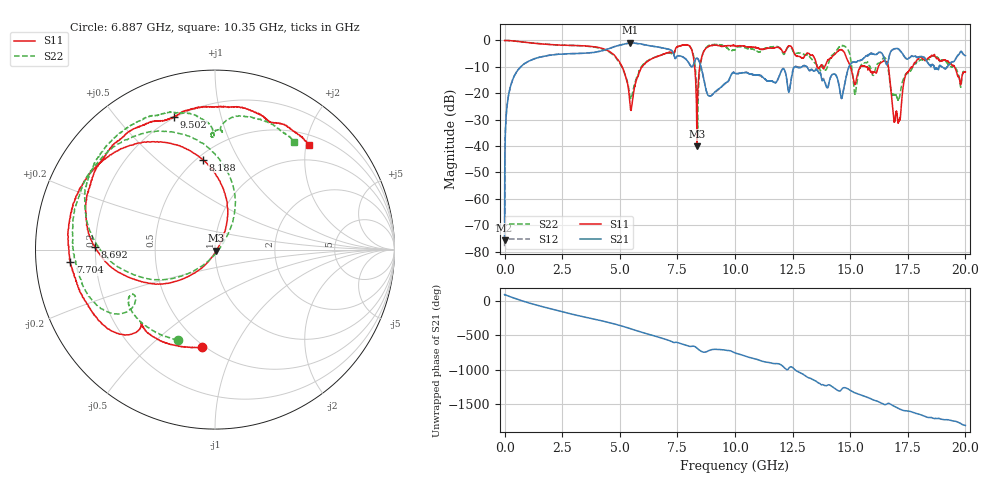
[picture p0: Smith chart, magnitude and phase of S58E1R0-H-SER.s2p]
!{S58E1R0}
!Johanson Technology Inc.
!www.johansontechnology.com
!Test Board Conditions:
!Substrate Type  RO4350B
!Substrate Thickness  60 mil
!Substrate Dk  3.66
!TL Type: GCPW
!TL Trace Width  115 mil
!TL Gap  52 mil
!Electrode orientation  Horizontal
!DUT TOPOLOGY	SERIES
!Mounting Pad LxW  55x428 mil
! Created Tue Apr 13 21:45:22 2021
# hz S ma R 50
! 2 Port Network Data from SP1.SP block
! freq  magS11  angS11  magS21  angS21  magS12  angS12  magS22  angS22
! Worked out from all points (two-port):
!   20001 points, 300 kHz to 20 GHz, reference 50 ohm
!   highest |S21| = -0.87 dB at 5.44 GHz (marker M1); lowest = -75.7 dB at 300 kHz (marker M2)
!   |S21| within 3 dB of the highest: 4.24 GHz to 7.264 GHz (3.024 GHz wide, 52.6 % of centre); 16.79 GHz to 17.17 GHz (381.5 MHz wide, 2.25 % of centre)
!   lowest |S11| = -40.1 dB at 8.347 GHz (marker M3), VSWR 1.02, Z = 50.8 - j0.539 ohm
!   |S11| at or under -10 dB: 5.105 GHz to 5.965 GHz (860.2 MHz wide, 15.5 % of centre); 16.66 GHz to 17.71 GHz (1.051 GHz wide, 6.12 % of centre); 19.53 GHz to end of sweep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
!   |S22| runs from -35.9 to 0.0 dB; largest |S21 - S12| = 0.013
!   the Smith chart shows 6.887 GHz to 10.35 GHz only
!   S11 on the Smith chart (normalised r, x): 6.887 GHz: 0.48, -0.75; 7.704 GHz: 0.11, -0.04; 8.188 GHz: 0.53, +0.72; 8.692 GHz: 0.20, +0.01; 9.502 GHz: 0.20, +0.72; 10.35 GHz: 0.69, +2.06
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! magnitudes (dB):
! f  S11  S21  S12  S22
! 300 kHz  0.0  -75.7  -77.9  -0.1
! 128.3 MHz  0.0  -23.2  -23.2  0.0
! 477.3 MHz  -0.3  -12.5  -12.5  -0.3
! 3.334 GHz  -2.0  -4.9  -4.9  -2.0
! 4.767 GHz  -5.6  -2.4  -2.3  -5.9
! 5.44 GHz  -24.1  -0.9  -0.9  -21.1
! 6.667 GHz  -6.0  -2.5  -2.5  -5.9
! 6.887 GHz  -5.2  -2.9  -2.9  -5.2
! 7.704 GHz  -1.8  -6.1  -6.1  -1.9
! 8.188 GHz  -5.9  -9.3  -9.5  -5.1
! 8.347 GHz  -40.1  -6.7  -6.8  -20.6
! 8.692 GHz  -3.5  -16.7  -16.5  -3.3
! 9.502 GHz  -2.2  -16.8  -16.8  -2.0
! 10 GHz  -2.0  -12.4  -12.4  -3.6
! 10.35 GHz  -2.1  -12.2  -12.2  -2.5
! 13.33 GHz  -5.5  -11.0  -11.0  -7.1
! 14.63 GHz  -3.5  -21.8  -21.9  -2.0
! 15.21 GHz  -16.6  -8.3  -8.2  -20.5
! 16.67 GHz  -10.4  -7.0  -7.1  -11.8
! 17.1 GHz  -30.8  -3.3  -3.3  -22.5
! 17.98 GHz  -6.7  -6.4  -6.2  -7.8
! 20 GHz  -11.9  -5.7  -5.7  -11.1
